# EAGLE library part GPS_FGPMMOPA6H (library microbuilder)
GPS Module - MTK MT3339 Chipset, -165dBm sensitivity, 22 channels, 10Hz, auto-select external antenna options
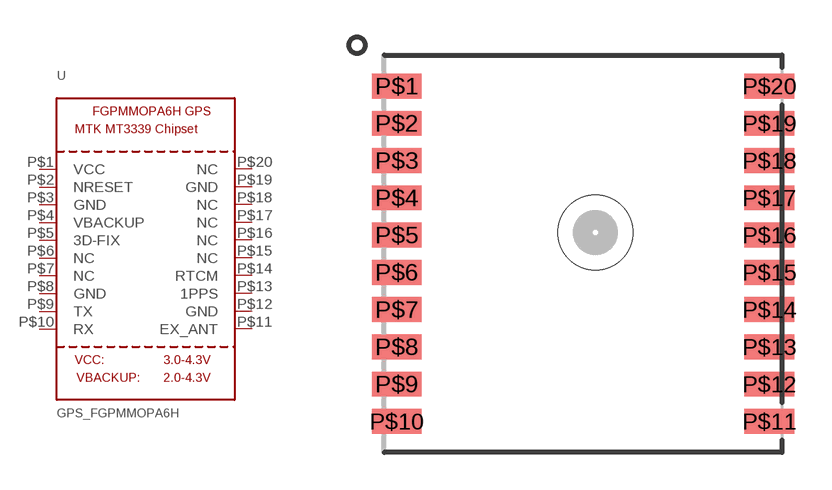
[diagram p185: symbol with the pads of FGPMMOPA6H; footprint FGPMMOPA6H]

Designator prefix U

## GPS_FGPMMOPA6H  [FGPMMOPA6H]
P$1  VCC
P$2  NRESET
P$3  GND
P$4  VBACKUP
P$5  3D-FIX
P$6  NC
P$7  NC
P$8  GND
P$9  TX
P$10  RX
P$11  EX_ANT
P$12  GND
P$13  1PPS
P$14  RTCM
P$15  NC
P$16  NC
P$17  NC
P$18  NC
P$19  GND
P$20  NC

## Footprint FGPMMOPA6H (pad centres in mm)
smd 2 x 1: P$1 -7.5,6.75; P$2 -7.5,5.25; P$3 -7.5,3.75; P$4 -7.5,2.25; P$5 -7.5,0.75; P$6 -7.5,-0.75; P$7 -7.5,-2.25; P$8 -7.5,-3.75; P$9 -7.5,-5.25; P$10 -7.5,-6.75; P$11 7.5,-6.75; P$12 7.5,-5.25; P$13 7.5,-3.75; P$14 7.5,-2.25; P$15 7.5,-0.75; P$16 7.5,0.75; P$17 7.5,2.25; P$18 7.5,3.75; P$19 7.5,5.25; P$20 7.5,6.75
hole 3 at 0.5,0.85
